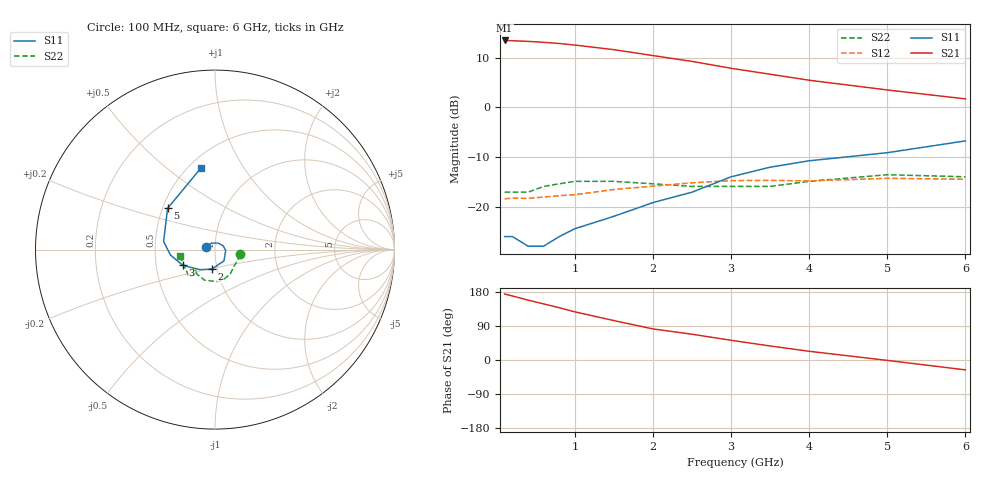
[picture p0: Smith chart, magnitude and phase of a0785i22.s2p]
!  MSA-0785 S AND NOISE PARAMETERS
!  Id=22mA  LAST UPDATED 07-27-92
# ghz s ma r 50
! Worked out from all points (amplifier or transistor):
!   14 points, 100 MHz to 6 GHz, reference 50 ohm
!   highest |S21| = 13.5 dB at 100 MHz (marker M1)
!   |S21| within 3 dB of that: start of sweep to 1.98 GHz
!   unconditionally stable (mu >= 1): start of sweep to end of sweep
!   at 400 MHz: K = 1.15, MAG = 13.5 dB, |S12| = -18.3 dB
!   at 2 GHz: K = 1.15, MAG = 10.8 dB, |S12| = -15.9 dB
!   at 6 GHz: K = 1.68, MAG = 3.3 dB, |S12| = -14.5 dB
!   lowest NFmin = 4.80 dB at 100 MHz
!   S11 on the Smith chart (normalised r, x): 100 MHz: 0.91, +0.02; 2 GHz: 0.94, -0.21; 3 GHz: 0.69, -0.13; 5 GHz: 0.53, +0.28; 6 GHz: 0.57, +0.66
0.1  0.05 166.0  4.73 174.0  0.12 1.0  0.14 -11.0
0.2  0.05 151.0  4.7 169.0  0.122 3.0  0.14 -21.0
0.4  0.04 115.0  4.63 158.0  0.121 6.0  0.14 -40.0
0.6  0.04 65.0  4.53 148.0  0.125 7.0  0.16 -58.0
0.8  0.05 26.0  4.41 138.0  0.129 9.0  0.17 -71.0
1  0.06 -5.0  4.25 127.0  0.132 10.0  0.18 -84.0
1.5  0.08 -51.0  3.82 104.0  0.149 12.0  0.18 -109.0
2  0.11 -99.0  3.33 82.0  0.161 11.0  0.17 -126.0
2.5  0.14 -127.0  2.91 68.0  0.174 13.0  0.16 -134.0
3  0.2 -154.0  2.48 52.0  0.183 7.0  0.16 -139.0
3.5  0.25 -173.0  2.16 37.0  0.184 5.0  0.16 -132.0
4  0.29 171.0  1.88 23.0  0.182 1.0  0.18 -130.0
5  0.35 139.0  1.5 -1.0  0.193 -6.0  0.21 -133.0
6  0.46 100.0  1.22 -26.0  0.189 -14.0  0.2 -169.0
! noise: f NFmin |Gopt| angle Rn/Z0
0.1  4.8  0.06  3  0.61
0.5  4.9  0.06  14  0.6
1  5  0.04  35  0.59
2  5.6  0.02  168  0.56
